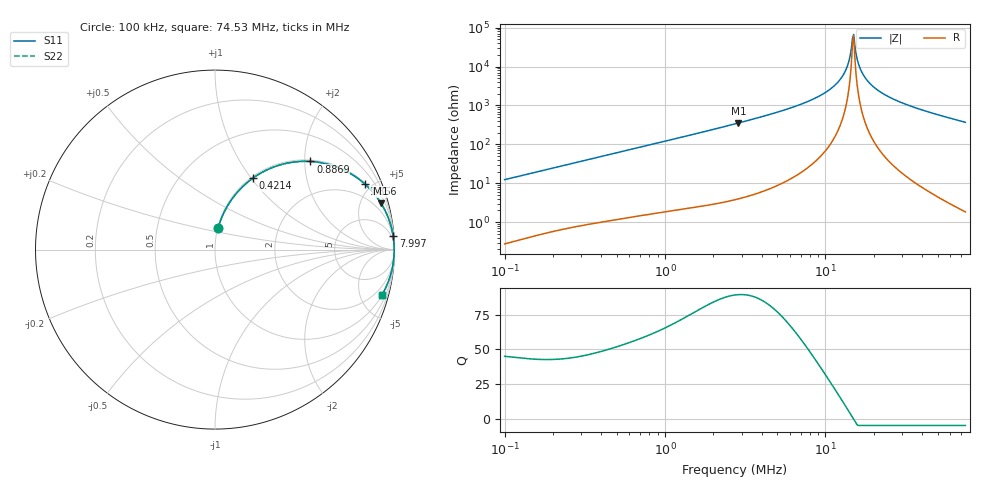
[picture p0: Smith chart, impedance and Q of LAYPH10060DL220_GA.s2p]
! LAYPH10060DL220_GA  S-PARAMETER MODEL  ( General Type )
! Model Generated by TAIYO YUDEN Corporation (http://www.ty-top.com)
! Version 3.0
! TAIYO YUDEN Control No. 180828NI43SB-FBB
! Copyright(c) 2017 TAIYO YUDEN CO.,LTD. All Rights Reserved.
! Product Description (link to TY-COMPAS)
! https://ds.yuden.co.jp/TYCOMPAS/or/detail?pn=LAYPH10060DL220MGA&u=M
! Products Name : Inductors
! Characteristics :
!  Inductance : 22 uH , SRF(min) : -Hz , DC Resistance(max) : 0.053 Ohm
!  Rated Current : Saturation :3.1 A , Temp Rise : 2.1 A (25 degC)
!  Case Size : 10.1 x 10.0 / 0.398 x 0.394 [mm/inch] , Thickness : 6 / 0.236 [mm/inch]
!  (Conditions: Temperature = 25 degC , DC Bias Current/Voltage = 0A / 0V)
! External Node Assignments :
!  1  o---GGG---o  2
! GND o---------o GND
! Frequency Range : 0.1MHz  -  74.526194MHz  [ 402 STEP ]
# MHz S RI R 50
! Freq[MHz].  S11 Real  S11 Imag  S21 Real  S21 Imag  S12 Real  S12 Imag  S22 Real  S22 Imag
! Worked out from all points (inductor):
!   401 points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, 100 kHz to 74.53 MHz, reference 50 ohm
!   read as one part in series: L = 19.6 uH near 103.4 kHz
!   highest Q = 89.4 at 2.869 MHz (marker M1), where L = 19.7 uH
!   self-resonance near 14.74 MHz
!   S11 on the Smith chart (normalised r, x): 100 kHz: 1.01, +0.25; 421.4 kHz: 1.02, +1.02; 886.9 kHz: 1.03, +2.13; 1.866 MHz: 1.05, +4.52; 7.997 MHz: 2, +27; 74.53 MHz: 1.04, -7.39
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0.1  0.0177 0.1213  0.9823 -0.1213  0.9823 -0.1213  0.0177 0.1213
0.302769  0.1248 0.3196  0.8752 -0.3196  0.8752 -0.3196  0.1248 0.3196
0.421432  0.2113 0.3981  0.7887 -0.3981  0.7887 -0.3981  0.2113 0.3981
0.886874  0.532 0.491  0.468 -0.491  0.468 -0.491  0.532 0.491
0.916692  0.5481 0.4898  0.4519 -0.4898  0.4519 -0.4898  0.5481 0.4898
1.866366  0.8334 0.3666  0.1666 -0.3666  0.1666 -0.3666  0.8334 0.3666
2.729949  0.9163 0.2714  0.0837 -0.2714  0.0837 -0.2714  0.9163 0.2714
2.868777  0.9239 0.2596  0.0761 -0.2596  0.0761 -0.2596  0.9239 0.2596
7.996587  0.9929 0.0743  0.00711 -0.0743  0.00711 -0.0743  0.9929 0.0743
8.265445  0.9935 0.0699  0.00646 -0.0699  0.00646 -0.0699  0.9935 0.0699
10.4183  0.9969 0.0411  0.00315 -0.0411  0.00315 -0.0411  0.9969 0.0411
12.2915  0.9981 0.0219  0.00189 -0.0219  0.00189 -0.0219  0.9981 0.0219
13.57342  0.9985 0.0106  0.0015 -0.0106  0.0015 -0.0106  0.9985 0.0106
14.50149  0.9986 0.00314  0.00139 -0.00314  0.00139 -0.00314  0.9986 0.00314
14.98905  0.9986 -0.000577  0.00138 0.000577  0.00138 0.000577  0.9986 -0.000577
15.23894  0.9986 -0.00244  0.00138 0.00244  0.00138 0.00244  0.9986 -0.00244
16.28088  0.9985 -0.00989  0.00146 0.00989  0.00146 0.00989  0.9985 -0.00989
17.68405  0.9983 -0.0193  0.00173 0.0193  0.00173 0.0193  0.9983 -0.0193
20.52148  0.9973 -0.0365  0.00268 0.0365  0.00268 0.0365  0.9973 -0.0365
25.02522  0.995 -0.0606  0.00503 0.0606  0.00503 0.0606  0.995 -0.0606
39.10739  0.983 -0.1241  0.017 0.1241  0.017 0.1241  0.983 -0.1241
74.52619  0.9307 -0.2514  0.0693 0.2514  0.0693 0.2514  0.9307 -0.2514
